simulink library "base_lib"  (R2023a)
settings: Solver=VariableStepAuto  StartTime=0.0  StopTime=10.0  RelTol=1e-3
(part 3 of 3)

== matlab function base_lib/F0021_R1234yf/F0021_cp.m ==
function cp = F0021_cp(T,rho)
%R1234yf_cp
%    CP = R1234yf_cp(T,RHO)

%    This function was generated by the Symbolic Math Toolbox version 9.3.
%    16-Oct-2023 15:47:52

t2 = rho.^2;
t3 = rho.^3;
t5 = rho.^5;
t7 = rho.^7;
t8 = 1.0./T;
t11 = rho./4.17e+3;
t16 = rho.*7.769784172661871e-3;
t24 = rho.*4.892086330935252e-4;
t29 = rho.*2.800959232613909e-3;
t31 = rho.*6.407673860911271e-4;
t32 = rho.*5.059952038369305e-4;
t4 = t2.^2;
t6 = t2.^3;
t9 = t8.^2;
t10 = t8.^3;
t12 = t8.*7.18e+2;
t13 = t8.*8.77e+2;
t14 = t8.*1.755e+3;
t15 = t8.*4.465e+3;
t17 = -t11;
t22 = t8.*5.8856e+4;
t30 = t8.*3.6785e+2;
t33 = t8.*7.94556e+4;
t34 = t2./1.73889e+7;
t39 = t8.*1.044694e+3;
t40 = t11-4.1e+1./2.5e+1;
t48 = t8.*6.54773e+2;
t49 = t8.*1.699467e+3;
t50 = t11-9.1e+1./1.0e+2;
t51 = t11-8.9e+1./1.25e+2;
t52 = t11-3.59e+2./5.0e+2;
t67 = t11-6.77e+2./1.0e+3;
t68 = t16-5.3136e+1;
t77 = t24-1.45248;
t86 = t29-8.38624;
t91 = t31-2.43152;
t99 = t32-1.42847;
t122 = t3.*t8.*9.319180196722149e-10;
t18 = -t12;
t19 = -t13;
t20 = -t14;
t21 = -t15;
t23 = exp(t17);
t41 = -t34;
t42 = t30.^(3.0./2.0);
t43 = t30.^(2.0./5.0);
t44 = t30.^(5.0./2.0);
t45 = t30.^(7.0./2.0);
t46 = t30.^(7.0./5.0);
t53 = t30-6.0./5.0;
t54 = t30.^(1.0./2.0e+1);
t55 = t40.^2;
t56 = t30.^(8.0./2.5e+1);
t58 = t30.^(1.9e+1./2.5e+1);
t60 = t30.^(3.6e+1./2.5e+1);
t61 = t30.^(1.9e+1./5.0e+1);
t62 = t30.^(4.4e+1./2.5e+1);
t64 = t30.^(6.1e+1./2.5e+1);
t65 = t30.^(4.7e+1./5.0e+1);
t66 = t22-2.048e+2;
t69 = t30-3.2e+1./2.5e+1;
t70 = t30-2.3e+1./5.0e+1;
t71 = 1.0./t30.^(3.0./1.0e+2);
t72 = t50.^2;
t73 = t51.^2;
t74 = t52.^2;
t76 = t30.^(9.7e+1./1.0e+2);
t78 = t30-6.7e+1./1.0e+2;
t79 = t30-1.13e+2./1.0e+2;
t80 = t33-2.592e+2;
t81 = t67.^2;
t84 = t30.^(9.29e+2./1.0e+3);
t96 = t39-3.2092;
t102 = t48-8.188e-1;
t105 = t49-3.0954;
t25 = exp(t18);
t26 = exp(t19);
t27 = exp(t20);
t28 = exp(t21);
t47 = exp(t41);
t57 = t54.^21;
t59 = t56.^4;
t63 = t58.^3;
t75 = t53.^2;
t82 = t69.^2;
t83 = t70.^2;
t87 = t78.^2;
t88 = t79.^2;
t89 = t55.*(8.1e+1./5.0);
t94 = t73.*(5.1e+1./5.0e+1);
t98 = t74.*(1.46e+2./2.5e+1);
t100 = t72.*(1.67e+2./1.25e+2);
t106 = t81.*(2.11e+2./2.0e+2);
t114 = t56.*1.546958;
t118 = t84.*2.355237;
t119 = rho.*t65.*2.315508393285372e-4;
t129 = t2.*t61.*3.033007263254145e-8;
t132 = rho.*t23.*t76.*3.263914628297362e-4;
t135 = t2.*t23.*t76.*3.913566700596357e-8;
t35 = t25-1.0;
t36 = t26-1.0;
t37 = t27-1.0;
t38 = t28-1.0;
t85 = t75.*1.08e+2;
t92 = -t89;
t93 = t82.*8.0e+1;
t97 = -t94;
t101 = -t98;
t103 = -t100;
t104 = t83.*(8.9e+1./1.0e+2);
t108 = t88.*(7.1e+1./5.0e+1);
t109 = -t106;
t111 = t87.*(2.31e+2./1.0e+2);
t120 = -t118;
t121 = -t119;
t130 = t47.*t63.*1.210006;
t133 = rho.*t47.*t64.*3.342232613908873e-4;
t136 = t2.*t47.*t63.*1.391699302428561e-7;
t137 = -t135;
t138 = t2.*t47.*t62.*1.06569432224005e-7;
t140 = t3.*t47.*t64.*1.922049476337705e-11;
t141 = t4.*t47.*t62.*4.085726420264459e-15;
t142 = t6.*t23.*t57.*3.588938332192827e-23;
t144 = t7.*t23.*t57.*1.229509534838242e-27;
t90 = -t85;
t95 = -t93;
t107 = -t104;
t110 = -t108;
t112 = -t111;
t131 = -t130;
t134 = -t133;
t139 = -t138;
t143 = -t142;
t113 = t90+t92;
t116 = t95+t101;
t123 = t97+t110;
t125 = t103+t112;
t126 = t107+t109;
t115 = exp(t113);
t117 = exp(t116);
t124 = exp(t123);
t127 = exp(t125);
t128 = exp(t126);
t145 = t2.*t8.*t117.*7.283294189396684e-5;
t147 = rho.*t45.*t115.*1.644384172661871e-7;
t148 = t46.*t124.*1.389966;
t149 = t10.*t127.*2.377824987227386e+7;
t151 = t2.*t45.*t128.*3.407663509480186e-8;
t153 = t3.*t8.*t86.*t117.*5.821977769301905e-9;
t154 = t2.*t45.*t68.*t115.*1.971683660266032e-11;
t156 = rho.*t46.*t77.*t124.*3.333251798561151e-4;
t158 = rho.*t10.*t91.*t127.*5.702218194789895e+3;
t159 = t3.*t45.*t99.*t128.*2.723951646267135e-12;
t146 = -t145;
t150 = -t149;
t152 = -t151;
t155 = -t154;
t157 = -t156;
t160 = t114+t120+t121+t122+t129+t131+t132+t134+t136+t137+t139+t140+t141+t143+t144+t146+t147+t148+t150+t152+t153+t155+t157+t158+t159;
et1 = 1.0./t35.^2.*exp(t8.*-1.436e+3).*2.876052391546904e+1+1.0./t36.^2.*exp(t8.*-1.754e+3).*8.736380352244283+1.0./t37.^2.*exp(t8.*-3.51e+3).*1.696916093943165e+2+1.0./t38.^2.*exp(t8.*-8.93e+3).*2.990869359808914e+2+rho.*t71.^56.*8.072375558752998e-5;
et2 = rho.*1.0./t30.^1.071.*(-3.72539753676259e-5)-(t25.*2.876052391546904e+1)./t35-(t26.*8.736380352244283)./t36-(t27.*1.696916093943165e+2)./t37-(t28.*2.990869359808914e+2)./t38;
et3 = t3.*t71.^54.*5.712042455816759e-13-t2.*1.0./t30.^(5.3e+1./5.0e+1).*1.565883373876438e-9+3.653734124219459e-5./t9+rho.*t30.^(7.0./2.5e+1).*t47.*8.468300984172661e-4;
et4 = rho.*1.0./t54.^12.*t124.*(-1.866621007194245e-4)+t7.*t23.*1.0./t54.^19.*6.454925057900768e-29+t2.*t30.^(1.1e+1./2.5e+1).*t47.*1.408065768852544e-7;
et5 = t3.*t47.*t71.^8.*1.139466607056987e-11+t2.*t23.*1.0./t30.^(1.03e+2./1.0e+2).*1.13884790987354e-9+rho.*t8.*t127.*2.528445291510791e-1;
et6 = rho.*t10.*t127.*(-2.634424805992931e+4)+rho.*t46.*t124.*9.466435107913669e-4-t3.*t8.*t117.*9.315164430883049e-7;
et7 = t2.*t42.*t115.*(-1.725223202732778e-10)+t2.*t45.*t115.*4.258836706174629e-9+t3.*t42.*t128.*2.383457690483743e-11-t3.*t45.*t128.*4.8486339303555e-12;
et8 = t3.*t66.*t117.*(-3.165408600952511e-11)-rho.*t9.*t105.*t127.*9.300886004822446e+1+rho.*t43.*t96.*t124.*9.333105035971223e-4+t2.*t44.*t80.*t115.*1.380178562186222e-10;
et9 = t3.*t44.*t102.*t128.*(-1.906766152386994e-11)+rho.*t10.*t105.^2.*t127.*5.702218194789895e+3-rho.*t46.*t96.^2.*t124.*3.333251798561151e-4;
et10 = t3.*t8.*t66.^2.*t117.*5.821977769301905e-9-t2.*t45.*t80.^2.*t115.*1.971683660266032e-11+t3.*t45.*t102.^2.*t128.*2.723951646267135e-12;
et11 = t65.*9.65567e-1+t137+t144-rho.*t61.*2.529528057553957e-4-t2.*t8.*1.165829442609941e-5-t23.*t76.*1.3610524;
et12 = t47.*t64.*1.393711-t45.*t115.*6.857082e-4+t86.*t153+t91.*t158+t99.*t159+rho.*t23.*t76.*6.527829256594724e-4+rho.*t47.*t62.*8.887890647482015e-4;
et13 = rho.*t47.*t63.*(-1.741015827338129e-3)+rho.*t8.*t117.*6.074267353956834e-1-rho.*t10.*t127.*1.52363270164786e+4+rho.*t46.*t124.*6.799833669064748e-4;
et14 = rho.*t45.*t128.*2.841991366906475e-4+t5.*t23.*t57.*8.979523707146454e-19-t6.*t23.*t57.*7.177876664385654e-23;
et15 = t3.*t47.*t62.*(-1.192623542075196e-10)-t2.*t47.*t64.*4.007473158164116e-7+t3.*t47.*t63.*6.674816798218516e-11+t5.*t47.*t62.*1.95958101691341e-18;
et16 = t4.*t47.*t64.*9.218462716247988e-15-t3.*t8.*t117.*6.800070034544626e-8+t2.*t45.*t115.*6.388255059261943e-10;
et17 = t3.*t45.*t128.*(-5.747537973623655e-12)-t10.*t91.*t127.*4.755649974454772e+7+t46.*t77.*t124.*2.779932+rho.*t45.*t68.*t115.*3.288768345323741e-7;
et18 = t2.*t8.*t86.*t117.*(-1.456658837879337e-4)-t2.*t45.*t99.*t128.*6.815327018960372e-8-rho.*t46.*t77.^2.*t124.*3.333251798561151e-4-t2.*t45.*t68.^2.*t115.*1.971683660266032e-11;
et19 = t3.*2.533418566459739e-12-t47.*t59.*2.75881368-t2.*t117.*1.979963079895795e-7-t9.*t127.*1.93923473200548e+5;
et20 = t43.*t124.*1.9459524+t66.*t145+t80.*t154+t96.*t156+t102.*t151+t105.*t149-rho.*t71.^2.*2.176577889688249e-4+t2.*1.0./t30.^(3.1e+1./5.0e+1).*1.152542760036575e-8+1.0./t30.^(1.7e+1./2.5e+1).*4.9502656e-1;
et21 = 1.0./t30.^(7.1e+1./1.0e+3).*(-2.188015173)+rho.*t23.*t71.*3.165997189448441e-4-rho.*t47.*t60.*8.155047577937649e-4+rho.*t44.*t115.*5.755344604316547e-7;
et22 = t6.*t23.*t54.*(-3.768385248802469e-23)+t7.*t23.*t54.*1.290985011580154e-27-t2.*t23.*t71.*3.796159699578467e-8;
et23 = t2.*t47.*t58.*(-1.875622007142488e-7)+t2.*t47.*t59.*3.173074409537118e-7+t4.*t47.*t58.*7.190878499665448e-15+t3.*t47.*t60.*4.689800722264001e-11;
et24 = t2.*t44.*t128.*(-1.192682228318065e-7)+t3.*t86.*t117.*1.582704300476255e-11-t46.*t96.*t124.*1.389966+rho.*t9.*t91.*t127.*4.650443002411223e+1;
et25 = rho.*t45.*t80.*t115.*(-1.644384172661871e-7)-rho.*t43.*t77.*t124.*4.666552517985612e-4-t2.*t44.*t68.*t115.*6.900892810931111e-11+t3.*t44.*t99.*t128.*9.533830761934972e-12;
et26 = rho.*t10.*t91.*t105.*t127.*(-5.702218194789895e+3)-t3.*t8.*t66.*t86.*t117.*5.821977769301905e-9-t3.*t45.*t99.*t102.*t128.*2.723951646267135e-12;
cp = t9.*(et1+et2+et3+et4+et5+et6+et7+et8+et9+et10).*1.12506132549482e+6+((t11.*t160-rho.*t8.*(et19+et20+et21+et22+et23+et24+et25+et26).*8.821342925659472e-2+1.0).^2.*8.314472)./((rho.*t160)./2.085e+3-(t2.*(et11+et12+et13+et14+et15+et16+et17+et18))./1.73889e+7+1.0);
end

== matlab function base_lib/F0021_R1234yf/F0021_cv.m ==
function cv = F0021_cv(T,rho)
%R1234yf_cv
%    CV = R1234yf_cv(T,RHO)

%    This function was generated by the Symbolic Math Toolbox version 9.3.
%    16-Oct-2023 15:47:50

t2 = rho.^2;
t3 = rho.^3;
t4 = 1.0./T;
t7 = rho./4.17e+3;
t5 = t4.^2;
t6 = t4.^3;
t8 = t4.*7.18e+2;
t9 = t4.*8.77e+2;
t10 = t4.*1.755e+3;
t11 = t4.*4.465e+3;
t12 = -t7;
t17 = t4.*5.8856e+4;
t23 = t4.*3.6785e+2;
t24 = t4.*7.94556e+4;
t25 = t2./1.73889e+7;
t30 = t4.*1.044694e+3;
t31 = t7-4.1e+1./2.5e+1;
t38 = t4.*6.54773e+2;
t39 = t4.*1.699467e+3;
t40 = t7-9.1e+1./1.0e+2;
t41 = t7-8.9e+1./1.25e+2;
t42 = t7-3.59e+2./5.0e+2;
t46 = t7-6.77e+2./1.0e+3;
t13 = -t8;
t14 = -t9;
t15 = -t10;
t16 = -t11;
t18 = exp(t12);
t32 = -t25;
t33 = t23.^(3.0./2.0);
t34 = t23.^(5.0./2.0);
t35 = t23.^(7.0./2.0);
t36 = t23.^(7.0./5.0);
t43 = t23-6.0./5.0;
t44 = t31.^2;
t45 = t17-2.048e+2;
t47 = t23-3.2e+1./2.5e+1;
t48 = t23-2.3e+1./5.0e+1;
t49 = t40.^2;
t50 = t41.^2;
t51 = t42.^2;
t53 = t23-6.7e+1./1.0e+2;
t54 = t23-1.13e+2./1.0e+2;
t55 = t24-2.592e+2;
t56 = t46.^2;
t68 = t30-3.2092;
t73 = t38-8.188e-1;
t76 = t39-3.0954;
t19 = exp(t13);
t20 = exp(t14);
t21 = exp(t15);
t22 = exp(t16);
t37 = exp(t32);
t52 = t43.^2;
t57 = t47.^2;
t58 = t48.^2;
t60 = t53.^2;
t61 = t54.^2;
t62 = t44.*(8.1e+1./5.0);
t66 = t50.*(5.1e+1./5.0e+1);
t70 = t51.*(1.46e+2./2.5e+1);
t71 = t49.*(1.67e+2./1.25e+2);
t77 = t56.*(2.11e+2./2.0e+2);
t26 = t19-1.0;
t27 = t20-1.0;
t28 = t21-1.0;
t29 = t22-1.0;
t59 = t52.*1.08e+2;
t64 = -t62;
t65 = t57.*8.0e+1;
t69 = -t66;
t72 = -t70;
t74 = -t71;
t75 = t58.*(8.9e+1./1.0e+2);
t79 = t61.*(7.1e+1./5.0e+1);
t80 = -t77;
t82 = t60.*(2.31e+2./1.0e+2);
t63 = -t59;
t67 = -t65;
t78 = -t75;
t81 = -t79;
t83 = -t82;
t84 = t63+t64;
t86 = t67+t72;
t88 = t69+t81;
t90 = t74+t83;
t91 = t78+t80;
t85 = exp(t84);
t87 = exp(t86);
t89 = exp(t88);
t92 = exp(t90);
t93 = exp(t91);
et1 = 1.0./t26.^2.*exp(t4.*-1.436e+3).*2.876052391546904e+1+1.0./t27.^2.*exp(t4.*-1.754e+3).*8.736380352244283+1.0./t28.^2.*exp(t4.*-3.51e+3).*1.696916093943165e+2+1.0./t29.^2.*exp(t4.*-8.93e+3).*2.990869359808914e+2+rho.*1.0./t23.^(4.2e+1./2.5e+1).*8.072375558752998e-5;
et2 = rho.*1.0./t23.^1.071.*(-3.72539753676259e-5)-(t19.*2.876052391546904e+1)./t26-(t20.*8.736380352244283)./t27-(t21.*1.696916093943165e+2)./t28-(t22.*2.990869359808914e+2)./t29;
et3 = t2.*1.0./t23.^(5.3e+1./5.0e+1).*(-1.565883373876438e-9)+t3.*1.0./t23.^(8.1e+1./5.0e+1).*5.712042455816759e-13+3.653734124219459e-5./t5+rho.*t23.^(7.0./2.5e+1).*t37.*8.468300984172661e-4;
et4 = rho.*1.0./t23.^(3.0./5.0).*t89.*(-1.866621007194245e-4)+t3.*1.0./t23.^(6.0./2.5e+1).*t37.*1.139466607056987e-11+t2.*t23.^(1.1e+1./2.5e+1).*t37.*1.408065768852544e-7;
et5 = t2.*t18.*1.0./t23.^(1.03e+2./1.0e+2).*1.13884790987354e-9+rho.^7.*t18.*1.0./t23.^(1.9e+1./2.0e+1).*6.454925057900768e-29+rho.*t4.*t92.*2.528445291510791e-1;
et6 = rho.*t6.*t92.*(-2.634424805992931e+4)+rho.*t36.*t89.*9.466435107913669e-4-t3.*t4.*t87.*9.315164430883049e-7;
et7 = t2.*t33.*t85.*(-1.725223202732778e-10)+t2.*t35.*t85.*4.258836706174629e-9+t3.*t33.*t93.*2.383457690483743e-11-t3.*t35.*t93.*4.8486339303555e-12;
et8 = t3.*t45.*t87.*(-3.165408600952511e-11)-rho.*t5.*t76.*t92.*9.300886004822446e+1+t2.*t34.*t55.*t85.*1.380178562186222e-10-t3.*t34.*t73.*t93.*1.906766152386994e-11;
et9 = rho.*t6.*t76.^2.*t92.*5.702218194789895e+3+rho.*t23.^(2.0./5.0).*t68.*t89.*9.333105035971223e-4-rho.*t36.*t68.^2.*t89.*3.333251798561151e-4;
et10 = t3.*t4.*t45.^2.*t87.*5.821977769301905e-9-t2.*t35.*t55.^2.*t85.*1.971683660266032e-11+t3.*t35.*t73.^2.*t93.*2.723951646267135e-12;
cv = t5.*(et1+et2+et3+et4+et5+et6+et7+et8+et9+et10).*1.12506132549482e+6;
end

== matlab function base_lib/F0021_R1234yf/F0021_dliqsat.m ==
function dliq = F0021_dliqsat(T)
% correlation from Martin (1959)


% critical Temp & density
Tc   =     367.85; % [K]
rhoc =     4170.0; % [mol/m3]

T = min(T, Tc);
T = max(T, 0);

% coefficients
x = [   1.768478200876913;
        0.905584244505430;
       -0.353914488877852;
        0.447866446078125 ];

% saturated liquid dfensity
Tr   = T ./ Tc;
A    = [ (1-Tr).^(1/3), (1-Tr).^(2/3), (1-Tr), (1-Tr).^(4/3) ];
dliq = rhoc .* ( 1 + A * x );


end

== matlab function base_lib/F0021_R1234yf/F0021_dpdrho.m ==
function dp_drho = R1234yf_dpdrho(T,rho)
%R1234yf_dpdrho
%    DP_DRHO = R1234yf_dpdrho(T,RHO)

%    This function was generated by the Symbolic Math Toolbox version 9.3.
%    27-Oct-2023 18:05:02

t2 = rho.^2;
t3 = rho.^3;
t5 = rho.^5;
t7 = rho.^7;
t8 = 1.0./T;
t10 = rho./4.17e+3;
t11 = rho.*7.769784172661871e-3;
t14 = rho.*4.892086330935252e-4;
t15 = rho.*2.800959232613909e-3;
t17 = rho.*6.407673860911271e-4;
t18 = rho.*5.059952038369305e-4;
t4 = t2.^2;
t6 = t2.^3;
t9 = t8.^3;
t12 = -t10;
t16 = t8.*3.6785e+2;
t19 = t2./1.73889e+7;
t20 = t10-4.1e+1./2.5e+1;
t25 = t10-9.1e+1./1.0e+2;
t26 = t10-8.9e+1./1.25e+2;
t27 = t10-3.59e+2./5.0e+2;
t36 = t10-6.77e+2./1.0e+3;
t37 = t11-5.3136e+1;
t45 = t14-1.45248;
t52 = t15-8.38624;
t57 = t17-2.43152;
t64 = t18-1.42847;
t13 = exp(t12);
t21 = -t19;
t22 = t16.^(7.0./2.0);
t23 = t16.^(7.0./5.0);
t28 = t16-6.0./5.0;
t29 = t20.^2;
t30 = t16.^(2.1e+1./2.0e+1);
t31 = t16.^(1.9e+1./5.0e+1);
t32 = t16.^(4.4e+1./2.5e+1);
t34 = t16.^(6.1e+1./2.5e+1);
t35 = t16.^(4.7e+1./5.0e+1);
t38 = t16-3.2e+1./2.5e+1;
t39 = t16-2.3e+1./5.0e+1;
t40 = t25.^2;
t41 = t26.^2;
t42 = t27.^2;
t44 = t16.^(9.7e+1./1.0e+2);
t46 = t16-6.7e+1./1.0e+2;
t47 = t16-1.13e+2./1.0e+2;
t48 = t36.^2;
t24 = exp(t21);
t33 = t31.^6;
t43 = t28.^2;
t49 = t38.^2;
t50 = t39.^2;
t53 = t46.^2;
t54 = t47.^2;
t55 = t29.*(8.1e+1./5.0);
t60 = t41.*(5.1e+1./5.0e+1);
t63 = t42.*(1.46e+2./2.5e+1);
t65 = t40.*(1.67e+2./1.25e+2);
t69 = t48.*(2.11e+2./2.0e+2);
t86 = t2.*t13.*t44.*3.913566700596357e-8;
t88 = t7.*t13.*t30.*1.229509534838242e-27;
t51 = t43.*1.08e+2;
t58 = -t55;
t59 = t49.*8.0e+1;
t62 = -t60;
t66 = -t63;
t67 = -t65;
t68 = t50.*(8.9e+1./1.0e+2);
t71 = t54.*(7.1e+1./5.0e+1);
t72 = -t69;
t74 = t53.*(2.31e+2./1.0e+2);
t87 = -t86;
t56 = -t51;
t61 = -t59;
t70 = -t68;
t73 = -t71;
t75 = -t74;
t76 = t56+t58;
t78 = t61+t66;
t80 = t62+t73;
t82 = t67+t75;
t83 = t70+t72;
t77 = exp(t76);
t79 = exp(t78);
t81 = exp(t80);
t84 = exp(t82);
t85 = exp(t83);
et1 = t87+t88-rho.*t35.*2.315508393285372e-4+t3.*t8.*9.319180196722149e-10+t2.*t31.*3.033007263254145e-8-t24.*t33.*1.210006;
et2 = t9.*t84.*(-2.377824987227386e+7)+t23.*t81.*1.389966+t16.^(8.0./2.5e+1).*1.546958-t16.^(9.29e+2./1.0e+3).*2.355237;
et3 = rho.*t13.*t44.*3.263914628297362e-4-rho.*t24.*t34.*3.342232613908873e-4+rho.*t22.*t77.*1.644384172661871e-7-t6.*t13.*t30.*3.588938332192827e-23;
et4 = t2.*t24.*t32.*(-1.06569432224005e-7)+t2.*t24.*t33.*1.391699302428561e-7+t4.*t24.*t32.*4.085726420264459e-15+t3.*t24.*t34.*1.922049476337705e-11;
et5 = t2.*t8.*t79.*(-7.283294189396684e-5)-t2.*t22.*t85.*3.407663509480186e-8-rho.*t23.*t45.*t81.*3.333251798561151e-4+rho.*t9.*t57.*t84.*5.702218194789895e+3;
et6 = t2.*t22.*t37.*t77.*(-1.971683660266032e-11)+t3.*t8.*t52.*t79.*5.821977769301905e-9+t3.*t22.*t64.*t85.*2.723951646267135e-12;
et7 = t35.*9.65567e-1+t87+t88-rho.*t31.*2.529528057553957e-4-t2.*t8.*1.165829442609941e-5-t13.*t44.*1.3610524;
et8 = t24.*t34.*1.393711-t22.*t77.*6.857082e-4+rho.*t24.*t32.*8.887890647482015e-4+rho.*t13.*t44.*6.527829256594724e-4-rho.*t24.*t33.*1.741015827338129e-3;
et9 = rho.*t8.*t79.*6.074267353956834e-1-rho.*t9.*t84.*1.52363270164786e+4+rho.*t23.*t81.*6.799833669064748e-4+rho.*t22.*t85.*2.841991366906475e-4;
et10 = t5.*t13.*t30.*8.979523707146454e-19-t6.*t13.*t30.*7.177876664385654e-23-t3.*t24.*t32.*1.192623542075196e-10;
et11 = t2.*t24.*t34.*(-4.007473158164116e-7)+t3.*t24.*t33.*6.674816798218516e-11+t5.*t24.*t32.*1.95958101691341e-18+t4.*t24.*t34.*9.218462716247988e-15;
et12 = t3.*t8.*t79.*(-6.800070034544626e-8)+t2.*t22.*t77.*6.388255059261943e-10-t3.*t22.*t85.*5.747537973623655e-12+t23.*t45.*t81.*2.779932;
et13 = t9.*t57.*t84.*(-4.755649974454772e+7)+rho.*t22.*t37.*t77.*3.288768345323741e-7-t2.*t8.*t52.*t79.*1.456658837879337e-4-t2.*t22.*t64.*t85.*6.815327018960372e-8;
et14 = rho.*t23.*t45.^2.*t81.*(-3.333251798561151e-4)+rho.*t9.*t57.^2.*t84.*5.702218194789895e+3-t2.*t22.*t37.^2.*t77.*1.971683660266032e-11;
et15 = t3.*t8.*t52.^2.*t79.*5.821977769301905e-9+t3.*t22.*t64.^2.*t85.*2.723951646267135e-12;
dp_drho = T.*((rho.*(et1+et2+et3+et4+et5+et6))./2.085e+3-(t2.*(et7+et8+et9+et10+et11+et12+et13+et14+et15))./1.73889e+7+1.0).*8.314472;
end

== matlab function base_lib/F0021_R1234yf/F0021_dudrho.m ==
function du_drho = R1234yf_dudrho(T,rho)
%R1234yf_dudrho
%    DU_DRHO = R1234yf_dudrho(T,RHO)

%    This function was generated by the Symbolic Math Toolbox version 9.3.
%    19-Oct-2023 14:13:06

t2 = rho.^2;
t3 = rho.^3;
t4 = 1.0./T;
t7 = rho./4.17e+3;
t12 = rho.*1.863257595362559e-6;
t15 = rho.*1.173162189672722e-7;
t19 = rho.*6.716928615381076e-7;
t20 = rho.*1.53661243666937e-7;
t21 = rho.*1.213417755004629e-7;
t5 = t4.^2;
t6 = t4.^3;
t8 = -t7;
t9 = t4.*5.8856e+4;
t11 = t4.*3.6785e+2;
t13 = t4.*7.94556e+4;
t14 = t2./1.73889e+7;
t16 = t4.*1.044694e+3;
t17 = t7-4.1e+1./2.5e+1;
t27 = t4.*6.54773e+2;
t28 = t4.*1.699467e+3;
t29 = t7-9.1e+1./1.0e+2;
t30 = t7-8.9e+1./1.25e+2;
t31 = t7-3.59e+2./5.0e+2;
t39 = t7-6.77e+2./1.0e+3;
t60 = t12-1.274244604316547e-2;
t68 = t15-3.483165467625899e-4;
t79 = t19-2.011088729016787e-3;
t81 = t20-5.830983213429257e-4;
t82 = t21-3.425587529976019e-4;
t10 = exp(t8);
t18 = -t14;
t22 = t11.^(2.0./5.0);
t23 = t11.^(5.0./2.0);
t24 = t11.^(7.0./2.0);
t25 = t11.^(7.0./5.0);
t32 = t11-6.0./5.0;
t33 = t11.^(1.0./2.0e+1);
t34 = t17.^2;
t35 = t11.^(1.9e+1./2.5e+1);
t36 = t11.^(3.2e+1./2.5e+1);
t37 = t11.^(3.6e+1./2.5e+1);
t38 = t9-2.048e+2;
t40 = t11-3.2e+1./2.5e+1;
t41 = t11-2.3e+1./5.0e+1;
t42 = 1.0./t11.^(3.0./1.0e+2);
t43 = t29.^2;
t44 = t30.^2;
t45 = t31.^2;
t47 = t11-6.7e+1./1.0e+2;
t48 = t11-1.13e+2./1.0e+2;
t49 = t13-2.592e+2;
t50 = t39.^2;
t63 = t16-3.2092;
t69 = t27-8.188e-1;
t72 = t28-3.0954;
t26 = exp(t18);
t46 = t32.^2;
t51 = t40.^2;
t52 = t41.^2;
t54 = t47.^2;
t55 = t48.^2;
t56 = t34.*(8.1e+1./5.0);
t61 = t44.*(5.1e+1./5.0e+1);
t65 = t45.*(1.46e+2./2.5e+1);
t66 = t43.*(1.67e+2./1.25e+2);
t73 = t50.*(2.11e+2./2.0e+2);
t53 = t46.*1.08e+2;
t58 = -t56;
t59 = t51.*8.0e+1;
t64 = -t61;
t67 = -t65;
t70 = -t66;
t71 = t52.*(8.9e+1./1.0e+2);
t75 = t55.*(7.1e+1./5.0e+1);
t76 = -t73;
t78 = t54.*(2.31e+2./1.0e+2);
t57 = -t53;
t62 = -t59;
t74 = -t71;
t77 = -t75;
t80 = -t78;
t83 = t57+t58;
t85 = t62+t67;
t87 = t64+t77;
t89 = t70+t80;
t90 = t74+t76;
t84 = exp(t83);
t86 = exp(t85);
t88 = exp(t87);
t91 = exp(t89);
t92 = exp(t90);
et1 = t3.*1.858131002604336e-12-t26.*t36.*2.023446617579852;
et2 = t2.*t86.*(-1.452200134424495e-7)-t5.*t91.*1.422328005554134e+5;
et3 = t22.*t88.*1.427255066297698-rho.*t42.^2.*1.59640689065627e-4;
et4 = t2.*1.0./t11.^(3.1e+1./5.0e+1).*8.453302832006239e-9+1.0./t11.^(1.7e+1./2.5e+1).*3.630762837322852e-1;
et5 = 1.0./t11.^(7.1e+1./1.0e+3).*(-1.60479554422836)+rho.^7.*t10.*t33.*9.468704878352454e-28;
et6 = t2.^3.*t10.*t33.*(-2.763914953991081e-23)+t2.^2.*t26.*t35.*5.274136083584932e-15;
et7 = rho.*t10.*t42.*2.322094583878085e-4-rho.*t26.*t37.*5.981304050145462e-4;
et8 = rho.*t23.*t84.*4.221246493387974e-7-t2.*t10.*t42.*2.784286071796265e-8;
et9 = t2.*t26.*t35.*(-1.37567137415775e-7)+t2.*t26.*t36.*2.327285357417493e-7;
et10 = t3.*t26.*t37.*3.439725370866163e-11-t2.*t23.*t92.*8.74770499448078e-8;
et11 = t3.*t79.*t86.*4.840667114748315e-8+t6.*t72.*t91.*1.74401118947696e+7;
et12 = t25.*t63.*t88.*(-1.019467904498356)-rho.*t24.*t49.*t84.*1.206070426682278e-7;
et13 = rho.*t5.*t81.*t91.*1.422328005554134e+5-rho.*t22.*t68.*t88.*1.427255066297698;
et14 = t2.*t4.*t38.*t86.*5.341918194480503e-5-t2.*t23.*t60.*t84.*2.110623246693987e-7;
et15 = t2.*t24.*t69.*t92.*2.499344284137366e-8+t3.*t23.*t82.*t92.*2.915901664826927e-8;
et16 = rho.*t25.*t63.*t68.*t88.*1.019467904498356-rho.*t6.*t72.*t81.*t91.*1.74401118947696e+7;
et17 = t3.*t4.*t38.*t79.*t86.*(-1.780639398160168e-5)+t2.*t24.*t49.*t60.*t84.*6.030352133411391e-8;
et18 = t3.*t24.*t69.*t82.*t92.*(-8.331147613791219e-9);
du_drho = et1+et2+et3+et4+et5+et6+et7+et8+et9+et10+et11+et12+et13+et14+et15+et16+et17+et18;
end

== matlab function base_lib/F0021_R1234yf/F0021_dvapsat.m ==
function dvap = F0021_dvapsat(T)

% critical Temp & density
Tc   =     367.85; % [K]
% rhoc =     4170.0; % [mol/m3]

T = min(T, Tc);
T = max(T, 0);

% coefficients
x = [ 8.5116; -7.9050; 1.6189; 2.6394; -1.3847 ];

% saturated vapor density
Tr   = T ./ Tc;
th   = 1 ./ (1 - Tr);
A    = [ ones(size(Tr)), log(th).^(-1.5), log(th).^(-2), log(th).^(-3), log(th).^(-4) ];
dvap = exp(A*x);


end

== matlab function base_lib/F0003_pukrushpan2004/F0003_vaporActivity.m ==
function a = F0003_vaporActivity(p, P_sat)
a = p ./ P_sat; % [-] - water vapor activity
end

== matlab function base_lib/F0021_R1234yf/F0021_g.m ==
function g = F0021_g(T,rho)
%R1234yf_g
%    G = R1234yf_g(T,RHO)

%    This function was generated by the Symbolic Math Toolbox version 9.3.
%    16-Oct-2023 15:47:52

t2 = rho.^2;
t3 = rho.^3;
t5 = rho.^7;
t6 = 1.0./T;
t8 = rho./4.17e+3;
t4 = t2.^2;
t7 = t6.^3;
t9 = -t8;
t11 = t6.*3.6785e+2;
t12 = t2./1.73889e+7;
t13 = t8-4.1e+1./2.5e+1;
t18 = t8-9.1e+1./1.0e+2;
t19 = t8-8.9e+1./1.25e+2;
t20 = t8-3.59e+2./5.0e+2;
t30 = t8-6.77e+2./1.0e+3;
t10 = exp(t9);
t14 = -t12;
t15 = t11.^(7.0./2.0);
t16 = t11.^(7.0./5.0);
t21 = t11-6.0./5.0;
t22 = t13.^2;
t23 = t11.^(8.0./2.5e+1);
t24 = t11.^(2.1e+1./2.0e+1);
t25 = t11.^(1.9e+1./5.0e+1);
t26 = t11.^(4.4e+1./2.5e+1);
t28 = t11.^(6.1e+1./2.5e+1);
t29 = t11.^(4.7e+1./5.0e+1);
t31 = t11-3.2e+1./2.5e+1;
t32 = t11-2.3e+1./5.0e+1;
t33 = t18.^2;
t34 = t19.^2;
t35 = t20.^2;
t37 = t11.^(9.7e+1./1.0e+2);
t38 = t11-6.7e+1./1.0e+2;
t39 = t11-1.13e+2./1.0e+2;
t40 = t30.^2;
t43 = t11.^(9.29e+2./1.0e+3);
t17 = exp(t14);
t27 = t25.^6;
t36 = t21.^2;
t41 = t31.^2;
t42 = t32.^2;
t45 = t38.^2;
t46 = t39.^2;
t47 = t22.*(8.1e+1./5.0);
t51 = t34.*(5.1e+1./5.0e+1);
t54 = t35.*(1.46e+2./2.5e+1);
t55 = t33.*(1.67e+2./1.25e+2);
t59 = t40.*(2.11e+2./2.0e+2);
t76 = t2.*t10.*t37.*3.913566700596357e-8;
t77 = t5.*t10.*t24.*1.229509534838242e-27;
t44 = t36.*1.08e+2;
t49 = -t47;
t50 = t41.*8.0e+1;
t53 = -t51;
t56 = -t54;
t57 = -t55;
t58 = t42.*(8.9e+1./1.0e+2);
t61 = t46.*(7.1e+1./5.0e+1);
t62 = -t59;
t64 = t45.*(2.31e+2./1.0e+2);
t48 = -t44;
t52 = -t50;
t60 = -t58;
t63 = -t61;
t65 = -t64;
t66 = t48+t49;
t68 = t52+t56;
t70 = t53+t63;
t72 = t57+t65;
t73 = t60+t62;
t67 = exp(t66);
t69 = exp(t68);
t71 = exp(t70);
t74 = exp(t72);
t75 = exp(t73);
et1 = t23.*1.546958-t43.*2.355237-t76+t77-rho.*t29.*2.315508393285372e-4+t3.*t6.*9.319180196722149e-10;
et2 = t2.*t25.*3.033007263254145e-8-t17.*t27.*1.210006-t7.*t74.*2.377824987227386e+7+t16.*t71.*1.389966;
et3 = t2.^3.*t10.*t24.*(-3.588938332192827e-23)-rho.*t17.*t28.*3.342232613908873e-4+rho.*t10.*t37.*3.263914628297362e-4+rho.*t15.*t67.*1.644384172661871e-7;
et4 = t2.*t17.*t26.*(-1.06569432224005e-7)+t2.*t17.*t27.*1.391699302428561e-7+t4.*t17.*t26.*4.085726420264459e-15+t3.*t17.*t28.*1.922049476337705e-11;
et5 = t2.*t6.*t69.*(-7.283294189396684e-5)-t2.*t15.*t75.*3.407663509480186e-8-rho.*t16.*t71.*(rho.*4.892086330935252e-4-1.45248).*3.333251798561151e-4;
et6 = rho.*t7.*t74.*(rho.*6.407673860911271e-4-2.43152).*5.702218194789895e+3-t2.*t15.*t67.*(rho.*7.769784172661871e-3-5.3136e+1).*1.971683660266032e-11;
et7 = t3.*t6.*t69.*(rho.*2.800959232613909e-3-8.38624).*5.821977769301905e-9+t3.*t15.*t75.*(rho.*5.059952038369305e-4-1.42847).*2.723951646267135e-12;
et8 = t6.*2.95847224925e+3+t76-t77+log(-exp(t6.*-7.18e+2)+1.0).*7.549+log(-exp(t6.*-8.77e+2)+1.0).*1.537+log(-exp(t6.*-1.755e+3)+1.0).*7.455+log(-exp(t6.*-4.465e+3)+1.0).*(2.03e+2./1.0e+2)+log(t8)+log(t11).*(6.18e+2./1.25e+2)+rho.*t23.*3.709731414868106e-4;
et9 = rho.*t43.*(-5.64805035971223e-4)+t4.*t6.*5.587038487243495e-14+t3.*t25.*2.424466237613225e-12-t2.*t29.*2.776388960773827e-8+t8.*(et1+et2+et3+et4+et5+et6+et7);
et10 = rho.*t17.*t27.*(-2.901693045563549e-4)-rho.*t7.*t74.*5.702218194789895e+3+rho.*t16.*t71.*3.333251798561151e-4-t3.*t17.*t26.*8.518739586251397e-12;
et11 = t2.*t17.*t28.*(-4.007473158164116e-8)-t3.*t6.*t69.*5.821977769301905e-9+t2.*t15.*t67.*1.971683660266032e-11-t3.*t15.*t75.*2.723951646267135e-12;
et12 = -1.1837928e+1;
g = T.*(et8+et9+et10+et11+et12).*8.314472;
end

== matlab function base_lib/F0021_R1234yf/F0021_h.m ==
function h = F0021_h(T,rho)
%R1234yf_h
%    H = R1234yf_h(T,RHO)

%    This function was generated by the Symbolic Math Toolbox version 9.3.
%    16-Oct-2023 15:47:51

t2 = rho.^2;
t3 = rho.^3;
t5 = rho.^7;
t6 = 1.0./T;
t8 = rho./4.17e+3;
t4 = t2.^2;
t7 = t6.^3;
t9 = t6.*7.18e+2;
t10 = t6.*8.77e+2;
t11 = t6.*1.755e+3;
t12 = t6.*4.465e+3;
t13 = -t8;
t23 = t6.*3.6785e+2;
t24 = t2./1.73889e+7;
t25 = t8-4.1e+1./2.5e+1;
t31 = t8-9.1e+1./1.0e+2;
t32 = t8-8.9e+1./1.25e+2;
t33 = t8-3.59e+2./5.0e+2;
t40 = t8-6.77e+2./1.0e+3;
t14 = -t9;
t15 = -t10;
t16 = -t11;
t17 = -t12;
t18 = exp(t13);
t26 = -t24;
t27 = t23.^(5.0./2.0);
t28 = t23.^(7.0./2.0);
t29 = t23.^(7.0./5.0);
t34 = t23-6.0./5.0;
t35 = t25.^2;
t36 = t23.^(2.1e+1./2.0e+1);
t37 = t23.^(4.4e+1./2.5e+1);
t38 = t23.^(5.7e+1./2.5e+1);
t39 = t23.^(6.1e+1./2.5e+1);
t41 = t23-3.2e+1./2.5e+1;
t42 = t23-2.3e+1./5.0e+1;
t43 = t31.^2;
t44 = t32.^2;
t45 = t33.^2;
t47 = t23.^(9.7e+1./1.0e+2);
t48 = t23-6.7e+1./1.0e+2;
t49 = t23-1.13e+2./1.0e+2;
t50 = t40.^2;
t19 = exp(t14);
t20 = exp(t15);
t21 = exp(t16);
t22 = exp(t17);
t30 = exp(t26);
t46 = t34.^2;
t51 = t41.^2;
t52 = t42.^2;
t54 = t48.^2;
t55 = t49.^2;
t56 = t35.*(8.1e+1./5.0);
t60 = t44.*(5.1e+1./5.0e+1);
t63 = t45.*(1.46e+2./2.5e+1);
t64 = t43.*(1.67e+2./1.25e+2);
t68 = t50.*(2.11e+2./2.0e+2);
t53 = t46.*1.08e+2;
t58 = -t56;
t59 = t51.*8.0e+1;
t62 = -t60;
t65 = -t63;
t66 = -t64;
t67 = t52.*(8.9e+1./1.0e+2);
t70 = t55.*(7.1e+1./5.0e+1);
t71 = -t68;
t73 = t54.*(2.31e+2./1.0e+2);
t57 = -t53;
t61 = -t59;
t69 = -t67;
t72 = -t70;
t74 = -t73;
t75 = t57+t58;
t77 = t61+t65;
t79 = t62+t72;
t81 = t66+t74;
t82 = t69+t71;
t76 = exp(t75);
t78 = exp(t77);
t80 = exp(t79);
t83 = exp(t81);
t84 = exp(t82);
et1 = T.*(-1.344026097594128e-2)-t4.*1.518836071019028e-16+(t19.*1.473476145167867e+1)./(t19-1.0)+(t20.*3.66439853201033)./(t20-1.0)+(t21.*3.556755470980019e+1)./(t21-1.0)+(t22.*2.464034253092293e+1)./(t22-1.0)+t3.*t78.*1.582704300476255e-11;
et2 = rho.*1.0./t23.^(1.7e+1./2.5e+1).*(-1.187114052757794e-4)+rho.*1.0./t23.^(7.1e+1./1.0e+3).*5.247038784172661e-4+t2.*1.0./t23.^(3.0./5.0e+1).*2.609805623127397e-8;
et3 = t3.*1.0./t23.^(3.1e+1./5.0e+1).*(-9.212971702930256e-13)+rho.*t6.^2.*t83.*4.650443002411223e+1-rho.*t23.^(2.0./5.0).*t80.*4.666552517985612e-4;
et4 = rho.*t23.^(3.2e+1./2.5e+1).*t30.*6.615860143884892e-4+t5.*t18.*t23.^(1.0./2.0e+1).*1.290985011580154e-27+t3.*t23.^(1.9e+1./2.5e+1).*t30.*1.499298167180246e-11;
et5 = t2.*t23.^(3.6e+1./2.5e+1).*t30.*9.778234505920443e-8-t2.*t18.*1.0./t23.^(3.0./1.0e+2).*3.796159699578467e-8-t2.*t27.*t76.*6.900892810931111e-11;
et6 = t3.*t27.*t84.*9.533830761934972e-12+rho.*t29.*t80.*(t6.*1.044694e+3-3.2092).*3.333251798561151e-4-rho.*t7.*t83.*(t6.*1.699467e+3-3.0954).*5.702218194789895e+3;
et7 = t3.*t6.*t78.*(t6.*5.8856e+4-2.048e+2).*(-5.821977769301905e-9)+t2.*t28.*t76.*(t6.*7.94556e+4-2.592e+2).*1.971683660266032e-11;
et8 = t3.*t28.*t84.*(t6.*6.54773e+2-8.188e-1).*(-2.723951646267135e-12)-8.042605;
et9 = t3.*t6.*9.319180196722149e-10-t30.*t38.*1.210006-t7.*t83.*2.377824987227386e+7+t29.*t80.*1.389966;
et10 = rho.*t23.^(4.7e+1./5.0e+1).*(-2.315508393285372e-4)+t2.*t23.^(1.9e+1./5.0e+1).*3.033007263254145e-8+t23.^(8.0./2.5e+1).*1.546958-t23.^(9.29e+2./1.0e+3).*2.355237;
et11 = t2.^3.*t18.*t36.*(-3.588938332192827e-23)+rho.*t18.*t47.*3.263914628297362e-4-rho.*t30.*t39.*3.342232613908873e-4+rho.*t28.*t76.*1.644384172661871e-7;
et12 = t5.*t18.*t36.*1.229509534838242e-27-t2.*t18.*t47.*3.913566700596357e-8-t2.*t30.*t37.*1.06569432224005e-7+t2.*t30.*t38.*1.391699302428561e-7;
et13 = t4.*t30.*t37.*4.085726420264459e-15+t3.*t30.*t39.*1.922049476337705e-11-t2.*t6.*t78.*7.283294189396684e-5-t2.*t28.*t84.*3.407663509480186e-8;
et14 = rho.*t29.*t80.*(rho.*4.892086330935252e-4-1.45248).*(-3.333251798561151e-4)+rho.*t7.*t83.*(rho.*6.407673860911271e-4-2.43152).*5.702218194789895e+3;
et15 = t2.*t28.*t76.*(rho.*7.769784172661871e-3-5.3136e+1).*(-1.971683660266032e-11)+t3.*t6.*t78.*(rho.*2.800959232613909e-3-8.38624).*5.821977769301905e-9;
et16 = t3.*t28.*t84.*(rho.*5.059952038369305e-4-1.42847).*2.723951646267135e-12;
h = T.*(t6.*(et1+et2+et3+et4+et5+et6+et7+et8).*(-3.6785e+2)+t8.*(et9+et10+et11+et12+et13+et14+et15+et16)+1.0).*8.314472;
end

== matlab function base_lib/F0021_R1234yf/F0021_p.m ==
function p = F0021_p(T,rho)
%R1234yf_p
%    P = R1234yf_p(T,RHO)

%    This function was generated by the Symbolic Math Toolbox version 9.3.
%    16-Oct-2023 15:47:49

t2 = rho.^2;
t3 = rho.^3;
t4 = 1.0./T;
t6 = rho./4.17e+3;
t5 = t4.^3;
t7 = -t6;
t9 = t4.*3.6785e+2;
t10 = t2./1.73889e+7;
t11 = t6-4.1e+1./2.5e+1;
t16 = t6-9.1e+1./1.0e+2;
t17 = t6-8.9e+1./1.25e+2;
t18 = t6-3.59e+2./5.0e+2;
t25 = t6-6.77e+2./1.0e+3;
t8 = exp(t7);
t12 = -t10;
t13 = t9.^(7.0./2.0);
t14 = t9.^(7.0./5.0);
t19 = t9-6.0./5.0;
t20 = t11.^2;
t21 = t9.^(2.1e+1./2.0e+1);
t22 = t9.^(4.4e+1./2.5e+1);
t23 = t9.^(5.7e+1./2.5e+1);
t24 = t9.^(6.1e+1./2.5e+1);
t26 = t9-3.2e+1./2.5e+1;
t27 = t9-2.3e+1./5.0e+1;
t28 = t16.^2;
t29 = t17.^2;
t30 = t18.^2;
t32 = t9.^(9.7e+1./1.0e+2);
t33 = t9-6.7e+1./1.0e+2;
t34 = t9-1.13e+2./1.0e+2;
t35 = t25.^2;
t15 = exp(t12);
t31 = t19.^2;
t36 = t26.^2;
t37 = t27.^2;
t39 = t33.^2;
t40 = t34.^2;
t41 = t20.*(8.1e+1./5.0);
t45 = t29.*(5.1e+1./5.0e+1);
t48 = t30.*(1.46e+2./2.5e+1);
t49 = t28.*(1.67e+2./1.25e+2);
t53 = t35.*(2.11e+2./2.0e+2);
t38 = t31.*1.08e+2;
t43 = -t41;
t44 = t36.*8.0e+1;
t47 = -t45;
t50 = -t48;
t51 = -t49;
t52 = t37.*(8.9e+1./1.0e+2);
t55 = t40.*(7.1e+1./5.0e+1);
t56 = -t53;
t58 = t39.*(2.31e+2./1.0e+2);
t42 = -t38;
t46 = -t44;
t54 = -t52;
t57 = -t55;
t59 = -t58;
t60 = t42+t43;
t62 = t46+t50;
t64 = t47+t57;
t66 = t51+t59;
t67 = t54+t56;
t61 = exp(t60);
t63 = exp(t62);
t65 = exp(t64);
t68 = exp(t66);
t69 = exp(t67);
et1 = t3.*t4.*9.319180196722149e-10-t15.*t23.*1.210006-t5.*t68.*2.377824987227386e+7+t14.*t65.*1.389966;
et2 = rho.*t9.^(4.7e+1./5.0e+1).*(-2.315508393285372e-4)+t2.*t9.^(1.9e+1./5.0e+1).*3.033007263254145e-8+t9.^(8.0./2.5e+1).*1.546958-t9.^(9.29e+2./1.0e+3).*2.355237;
et3 = rho.^7.*t8.*t21.*1.229509534838242e-27-t2.^3.*t8.*t21.*3.588938332192827e-23+t2.^2.*t15.*t22.*4.085726420264459e-15;
et4 = rho.*t15.*t24.*(-3.342232613908873e-4)+rho.*t8.*t32.*3.263914628297362e-4+rho.*t13.*t61.*1.644384172661871e-7-t2.*t15.*t22.*1.06569432224005e-7;
et5 = t2.*t15.*t23.*1.391699302428561e-7-t2.*t8.*t32.*3.913566700596357e-8+t3.*t15.*t24.*1.922049476337705e-11-t2.*t4.*t63.*7.283294189396684e-5;
et6 = t2.*t13.*t69.*(-3.407663509480186e-8)-rho.*t14.*t65.*(rho.*4.892086330935252e-4-1.45248).*3.333251798561151e-4+rho.*t5.*t68.*(rho.*6.407673860911271e-4-2.43152).*5.702218194789895e+3;
et7 = t2.*t13.*t61.*(rho.*7.769784172661871e-3-5.3136e+1).*(-1.971683660266032e-11)+t3.*t4.*t63.*(rho.*2.800959232613909e-3-8.38624).*5.821977769301905e-9;
et8 = t3.*t13.*t69.*(rho.*5.059952038369305e-4-1.42847).*2.723951646267135e-12;
p = T.*rho.*(t6.*(et1+et2+et3+et4+et5+et6+et7+et8)+1.0).*8.314472;
end

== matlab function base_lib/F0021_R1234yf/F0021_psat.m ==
function p_sat = F0021_psat(T)
% Van Laar, J. L Res Tray Chim 39 (1920) 21
% fit to data from 
% Richter, Mclinden, Lemmon Journal of. Chem. E (2011)

% critical Temp & density
Tc   =     367.85; % [K]

T = max(T,0);
T = min(T, Tc);


% R1234yf coefficients
n = [ -4.893666065312787; 
       0.111013414194105; 
       0.000025221844863;
       -0.015565681357114] * 1e3;

% saturation pressure
p_sat = exp( n(1) .* (1./T) + n(2) + n(3) .* T + n(4) .* log(T) ); 
end

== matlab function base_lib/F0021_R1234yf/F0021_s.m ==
function s = F0021_s(T,rho)
%R1234yf_s
%    S = R1234yf_s(T,RHO)

%    This function was generated by the Symbolic Math Toolbox version 9.3.
%    16-Oct-2023 15:47:49

t2 = rho.^2;
t3 = rho.^3;
t5 = rho.^7;
t6 = 1.0./T;
t8 = rho./4.17e+3;
t4 = t2.^2;
t7 = t6.^3;
t9 = t6.*7.18e+2;
t10 = t6.*8.77e+2;
t11 = t6.*1.755e+3;
t12 = t6.*4.465e+3;
t13 = -t8;
t23 = t6.*3.6785e+2;
t24 = t2./1.73889e+7;
t25 = t8-4.1e+1./2.5e+1;
t31 = t8-9.1e+1./1.0e+2;
t32 = t8-8.9e+1./1.25e+2;
t33 = t8-3.59e+2./5.0e+2;
t36 = t8-6.77e+2./1.0e+3;
t14 = -t9;
t15 = -t10;
t16 = -t11;
t17 = -t12;
t18 = exp(t13);
t26 = -t24;
t27 = t23.^(5.0./2.0);
t28 = t23.^(7.0./2.0);
t29 = t23.^(7.0./5.0);
t34 = t23-6.0./5.0;
t35 = t25.^2;
t37 = t23-3.2e+1./2.5e+1;
t38 = t23-2.3e+1./5.0e+1;
t39 = t31.^2;
t40 = t32.^2;
t41 = t33.^2;
t43 = t23-6.7e+1./1.0e+2;
t44 = t23-1.13e+2./1.0e+2;
t45 = t36.^2;
t19 = exp(t14);
t20 = exp(t15);
t21 = exp(t16);
t22 = exp(t17);
t30 = exp(t26);
t42 = t34.^2;
t46 = t37.^2;
t47 = t38.^2;
t49 = t43.^2;
t50 = t44.^2;
t51 = t35.*(8.1e+1./5.0);
t55 = t40.*(5.1e+1./5.0e+1);
t58 = t41.*(1.46e+2./2.5e+1);
t59 = t39.*(1.67e+2./1.25e+2);
t63 = t45.*(2.11e+2./2.0e+2);
t48 = t42.*1.08e+2;
t53 = -t51;
t54 = t46.*8.0e+1;
t57 = -t55;
t60 = -t58;
t61 = -t59;
t62 = t47.*(8.9e+1./1.0e+2);
t65 = t50.*(7.1e+1./5.0e+1);
t66 = -t63;
t68 = t49.*(2.31e+2./1.0e+2);
t52 = -t48;
t56 = -t54;
t64 = -t62;
t67 = -t65;
t69 = -t68;
t70 = t52+t53;
t72 = t56+t60;
t74 = t57+t67;
t76 = t61+t69;
t77 = t64+t66;
t71 = exp(t70);
t73 = exp(t72);
t75 = exp(t74);
t78 = exp(t76);
t79 = exp(t77);
et1 = T.*(-1.344026097594128e-2)-t4.*1.518836071019028e-16+(t19.*1.473476145167867e+1)./(t19-1.0)+(t20.*3.66439853201033)./(t20-1.0)+(t21.*3.556755470980019e+1)./(t21-1.0)+(t22.*2.464034253092293e+1)./(t22-1.0)+t3.*t73.*1.582704300476255e-11;
et2 = rho.*1.0./t23.^(1.7e+1./2.5e+1).*(-1.187114052757794e-4)+rho.*1.0./t23.^(7.1e+1./1.0e+3).*5.247038784172661e-4+t2.*1.0./t23.^(3.0./5.0e+1).*2.609805623127397e-8;
et3 = t3.*1.0./t23.^(3.1e+1./5.0e+1).*(-9.212971702930256e-13)+rho.*t6.^2.*t78.*4.650443002411223e+1-rho.*t23.^(2.0./5.0).*t75.*4.666552517985612e-4;
et4 = rho.*t23.^(3.2e+1./2.5e+1).*t30.*6.615860143884892e-4+t5.*t18.*t23.^(1.0./2.0e+1).*1.290985011580154e-27+t3.*t23.^(1.9e+1./2.5e+1).*t30.*1.499298167180246e-11;
et5 = t2.*t23.^(3.6e+1./2.5e+1).*t30.*9.778234505920443e-8-t2.*t18.*1.0./t23.^(3.0./1.0e+2).*3.796159699578467e-8-t2.*t27.*t71.*6.900892810931111e-11;
et6 = t3.*t27.*t79.*9.533830761934972e-12+rho.*t29.*t75.*(t6.*1.044694e+3-3.2092).*3.333251798561151e-4-rho.*t7.*t78.*(t6.*1.699467e+3-3.0954).*5.702218194789895e+3;
et7 = t3.*t6.*t73.*(t6.*5.8856e+4-2.048e+2).*(-5.821977769301905e-9)+t2.*t28.*t71.*(t6.*7.94556e+4-2.592e+2).*1.971683660266032e-11;
et8 = t3.*t28.*t79.*(t6.*6.54773e+2-8.188e-1).*(-2.723951646267135e-12)-8.042605;
et9 = t6.*(-2.459813467916615e+4)-log(-t19+1.0).*6.2765949128e+1-log(-t20+1.0).*1.2779343464e+1;
et10 = log(-t21+1.0).*(-6.198438876e+1)-log(-t22+1.0).*1.687837816e+1-log(t8).*8.314472-log(t23).*4.1106749568e+1;
et11 = t4.*t6.*(-4.64532750651084e-13)-t6.*(et1+et2+et3+et4+et5+et6+et7+et8).*3.0584785252e+3;
et12 = rho.*t23.^(8.0./2.5e+1).*(-3.084445797644125e-3)+rho.*t23.^(9.29e+2./1.0e+3).*4.696055657041726e-3;
et13 = t3.*t23.^(1.9e+1./5.0e+1).*(-2.015815664758051e-11)+t2.*t23.^(4.7e+1./5.0e+1).*2.308420827546308e-7;
et14 = rho.*t23.^(5.7e+1./2.5e+1).*t30.*2.412604557993285e-3+t5.*t18.*t23.^(2.1e+1./2.0e+1).*1.022272260114558e-26;
et15 = t3.*t23.^(4.4e+1./2.5e+1).*t30.*7.082882176517883e-11+t2.*t23.^(6.1e+1./2.5e+1).*t30.*3.332002336430711e-7;
et16 = t2.*t18.*t23.^(9.7e+1./1.0e+2).*(-3.25392407522408e-7)+rho.*t7.*t78.*4.741093351847113e+4;
et17 = rho.*t29.*t75.*(-2.771422874808633e-3)+t3.*t6.*t73.*4.840667114748315e-8;
et18 = t2.*t28.*t71.*(-1.639350858613943e-10)+t3.*t28.*t79.*2.2648219692242e-11;
et19 = 1.06740592894016e+2;
s = et9+et10+et11+et12+et13+et14+et15+et16+et17+et18+et19;
end

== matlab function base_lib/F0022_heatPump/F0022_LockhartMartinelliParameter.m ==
function X_tt = F0022_LockhartMartinelliParameter(x, rho_g, rho_f, mu_g, mu_f)

% Lockhart-Martinelly Parameter (nuclear-power.com)
X_tt = ((1-x)./x).^0.9 .* (rho_g ./ rho_f).^0.5 .* (mu_f ./ mu_g ).^0.1;


end

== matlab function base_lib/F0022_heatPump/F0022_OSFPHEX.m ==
function h = F0022_OSFPHEX(G, x, rho_f, rho_g, cp_f, cp_g, mu_f, mu_g, k_f, k_g, sigma, par)

% parameters
D_h = par.D_h;

% output size
h = zeros(size(x));

% Bond number
g   = 9.81;
B_d = g .* (rho_f - rho_g) .* D_h.^2 ./ sigma;

% liquid & gas Prandtl number
Pr_f = cp_f .* mu_f ./ k_f;
Pr_g = cp_g .* mu_g ./ k_g;

% minimum mass flux
G = max(G, 1);

% refrigerant side heat transfer coefficient
G_eq  = G .* ( (1-x) + (rho_f./rho_g).^0.5 .* x );
Re_f  = G    .* D_h ./ mu_f;
Re_g  = G    .* D_h ./ mu_g;
Re_eq = G_eq .* D_h ./ mu_f;
Nu    = 3.918 .* Re_eq.^0.505 .* Re_f.^(-0.1354) .* B_d.^0.213 .* Pr_f.^(1/3);
h_tp     = Nu .* k_f ./ D_h;

% single phase correlation
h_f = 0.494 .* G .* cp_f .* Re_f.^(-0.426) .* Pr_f.^(-2/3);
h_g = 0.494 .* G .* cp_g .* Re_g.^(-0.426) .* Pr_g.^(-2/3);

% smooth transition to subcooled liquid & superheated vapor
y = (x-0.1) / 0.1;
y = tanh(y*5)/2 + 1/2;
z =  (x-0.90) / 0.1;
z = tanh(z*5)/2 + 1/2;

h = h_tp .* y .* (1-z) + h_f .* (1-y) + h_g .* z;

% output
% h       = h_tp;
% h(x==0) = h_f(x==0);
% h(x==1) = h_g(x==1);



end

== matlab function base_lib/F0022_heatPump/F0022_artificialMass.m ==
function m = F0022_artificialMass(p, par)

% parameters
B       = par.BV .* par.V;
rho_ref = par.rho_ref;
V       = par.V;

% artificial mass
m = V .* rho_ref .* (p./B + 1);


end

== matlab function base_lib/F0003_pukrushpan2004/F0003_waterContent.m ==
function lambda = F0003_waterContent(a)
lambda = zeros(length(a),1);
lambda( a <= 1) = 0.043 + 17.81.*a - 39.85.*a.^2 + 36.*a.^3;
lambda( a > 1)  = 14 + 1.4*(a-1);
end

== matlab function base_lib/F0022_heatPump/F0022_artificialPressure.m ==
function p = F0022_artificialPressure(m, par)

% parameters
V = par.V;
B = par.BV .* par.V;
rho_ref = par.rho_ref;


% artificial pressure
p = B .* (m./(V .* rho_ref) - 1); 

end

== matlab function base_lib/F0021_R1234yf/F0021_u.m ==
function u = F0021_u(T,rho)
%R1234yf_u
%    U = R1234yf_u(T,RHO)

%    This function was generated by the Symbolic Math Toolbox version 9.3.
%    16-Oct-2023 15:47:50

t2 = rho.^2;
t3 = rho.^3;
t4 = 1.0./T;
t5 = rho./4.17e+3;
t6 = t4.*7.18e+2;
t7 = t4.*8.77e+2;
t8 = t4.*1.755e+3;
t9 = t4.*4.465e+3;
t10 = -t5;
t20 = t4.*3.6785e+2;
t21 = t2./1.73889e+7;
t22 = t5-4.1e+1./2.5e+1;
t27 = t5-9.1e+1./1.0e+2;
t28 = t5-8.9e+1./1.25e+2;
t29 = t5-3.59e+2./5.0e+2;
t32 = t5-6.77e+2./1.0e+3;
t11 = -t6;
t12 = -t7;
t13 = -t8;
t14 = -t9;
t15 = exp(t10);
t23 = -t21;
t24 = t20.^(5.0./2.0);
t25 = t20.^(7.0./2.0);
t30 = t20-6.0./5.0;
t31 = t22.^2;
t33 = t20-3.2e+1./2.5e+1;
t34 = t20-2.3e+1./5.0e+1;
t35 = t27.^2;
t36 = t28.^2;
t37 = t29.^2;
t39 = t20-6.7e+1./1.0e+2;
t40 = t20-1.13e+2./1.0e+2;
t41 = t32.^2;
t16 = exp(t11);
t17 = exp(t12);
t18 = exp(t13);
t19 = exp(t14);
t26 = exp(t23);
t38 = t30.^2;
t42 = t33.^2;
t43 = t34.^2;
t45 = t39.^2;
t46 = t40.^2;
t47 = t31.*(8.1e+1./5.0);
t51 = t36.*(5.1e+1./5.0e+1);
t54 = t37.*(1.46e+2./2.5e+1);
t55 = t35.*(1.67e+2./1.25e+2);
t59 = t41.*(2.11e+2./2.0e+2);
t44 = t38.*1.08e+2;
t49 = -t47;
t50 = t42.*8.0e+1;
t53 = -t51;
t56 = -t54;
t57 = -t55;
t58 = t43.*(8.9e+1./1.0e+2);
t61 = t46.*(7.1e+1./5.0e+1);
t62 = -t59;
t64 = t45.*(2.31e+2./1.0e+2);
t48 = -t44;
t52 = -t50;
t60 = -t58;
t63 = -t61;
t65 = -t64;
t66 = t48+t49;
t68 = t52+t56;
t70 = t53+t63;
t72 = t57+t65;
t73 = t60+t62;
t67 = exp(t66);
t69 = exp(t68);
t71 = exp(t70);
t74 = exp(t72);
t75 = exp(t73);
et1 = T.*4.1106749568e+1-(t16.*4.5065951473904e+4)./(t16-1.0)-(t17.*1.1207484217928e+4)./(t17-1.0)-(t18.*1.087826022738e+5)./(t18-1.0);
et2 = (t19.*(-7.53619584844e+4))./(t19-1.0)-t3.*t69.*4.840667114748315e-8;
et3 = rho.*1.0./t20.^(1.7e+1./2.5e+1).*3.630762837322852e-1-rho.*1.0./t20.^(7.1e+1./1.0e+3).*1.60479554422836;
et4 = t2.*1.0./t20.^(3.0./5.0e+1).*(-7.982034453281349e-5)+t3.*1.0./t20.^(3.1e+1./5.0e+1).*2.817767610668746e-9;
et5 = t2.^2.*4.64532750651084e-13-rho.*t4.^2.*t74.*1.422328005554134e+5;
et6 = rho.*t20.^(2.0./5.0).*t71.*1.427255066297698-rho.*t20.^(3.2e+1./2.5e+1).*t26.*2.023446617579852;
et7 = t3.*t20.^(1.9e+1./2.5e+1).*t26.*(-4.585571247192502e-8)-t2.*t20.^(3.6e+1./2.5e+1).*t26.*2.990652025072731e-4;
et8 = t2.*t15.*1.0./t20.^(3.0./1.0e+2).*1.161047291939042e-4-rho.^7.*t15.*t20.^(1.0./2.0e+1).*3.948449934272973e-24;
et9 = t2.*t24.*t67.*2.110623246693987e-7-t3.*t24.*t75.*2.915901664826927e-8;
et10 = rho.*t20.^(7.0./5.0).*t71.*(t4.*1.044694e+3-3.2092).*(-1.019467904498356);
et11 = rho.*t4.^3.*t74.*(t4.*1.699467e+3-3.0954).*1.74401118947696e+7;
et12 = t3.*t4.*t69.*(t4.*5.8856e+4-2.048e+2).*1.780639398160168e-5-t2.*t25.*t67.*(t4.*7.94556e+4-2.592e+2).*6.030352133411391e-8;
et13 = t3.*t25.*t75.*(t4.*6.54773e+2-8.188e-1).*8.331147613791219e-9+2.459813467916615e+4;
u = et1+et2+et3+et4+et5+et6+et7+et8+et9+et10+et11+et12+et13;
end

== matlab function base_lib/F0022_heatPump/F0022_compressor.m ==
function [m_dot, P_cmp, h_2]  = F0022_compressor(p_1, rho_1, h_1, p_2, N, k, par)
% model from Li 2013

% parameters
V_disp = par.V_disp; 
N_ref  = par.N_ref / 60;
M      = par.M;

% M = 0.1140415928; % [kg/mol]  compressor displacement
% V_disp = 0.00017; % [m3]   compressor displacement
% N_ref = 2000 / 60; % [rps]  reference speed

% suction properties
p_s   = p_1;
rho_s = rho_1;
h_s   = h_1;

% discharge properties
p_d = p_2;

% compressor parameters
b1    = 0.799;
b2    = -0.036;
a1    = 1.140;
a2    = 0.295;
a3    = 447.050;
Wloss = 350.000;
d1    = 1.223;
d2    = -0.206;
d3    = -0.017;
e1    = 0.507;
e2    = 0.606;
e3    = -0.113;

% reference volumetric efficieny
nv_ref = b1 + b2 .* (  (p_d./p_s ).^(1./k) );

% reference volume flow
dV_ref = nv_ref .* N_ref .* V_disp;

% reference compressor power
P_ref = p_s .* dV_ref .* a1 .* ( (p_d./p_s).^(a2 + (k-1)./k) + a3./p_d ) + Wloss; 

% volumetric efficiency ratio
nv = d1 + d2 .* (N./N_ref) + d3 .* (N./N_ref).^2;

% isentropic efficiency ratio
ni = e1 + e2 .* (N./N_ref) + e3 .* (N./N_ref).^2; 

% Compressor suction volume flow
dV_suc = dV_ref .* (N./N_ref) .* nv;
m_dot  = dV_suc  .* rho_s .* M;

% Compressor power
P_cmp = P_ref .* dV_suc ./ dV_ref .* ni;

% discharge enthalpy
h_d = M.* P_cmp ./ (m_dot + 1e-5) + h_s;
h_2 = h_d;

end

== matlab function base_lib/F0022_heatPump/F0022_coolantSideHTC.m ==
function h = F0022_coolantSideHTC(G, par)
% parameters
mu = par.mu_clt;
k  = par.k_clt;
cp = par.cp_clt;

G = max(1,G);

% hydraulic diameter
D_h = par.D_h;

% Reynolds number
Re = G .* D_h ./ mu;

% Prandtl number
Pr = cp .* mu ./ k;

% HTC
h = 0.494 .* G .* cp .* Re.^(-0.426) .* Pr.^(-2/3);

end

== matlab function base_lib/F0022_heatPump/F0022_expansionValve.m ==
function dp = F0022_expansionValve(W, p_us, T_us, rho_us, T_sat, alpha, par)

% parameters
M  = par.M;
Tc = par.Tc;
D  = par.D;

% constants
R = 8.314472;

% exv geometry
A = alpha .* D.^2 .* pi / 4;

% degree of subcooling
T_sub = max(T_sat - T_us, 0);

% flow coefficient
a  = [ 0.7568; -1.7428; 1.0530; 2.2342; 2.9406;  -8.4168 ];
AA = [ones(size(p_us)), alpha, alpha.^2, alpha .* T_sub/Tc, T_sub/Tc,  (T_sub/Tc).^2 ];
C  = AA * a;

% pressure drop
dp =  1./rho_us .*  (W ./ (C.*A)).^2;


% pressure drop
% dp = p_us - p_ds;

% flow
% W = C.*A .* sqrt( rho_us .* max(dp,0) );

end

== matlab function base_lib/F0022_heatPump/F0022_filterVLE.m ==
function B = F0022_filterVLE(B, B_liq, B_vap, x)

% assign saturated property
B( x > 0 & x < 1) = x .* B_vap + (1-x) .* B_liq;


end

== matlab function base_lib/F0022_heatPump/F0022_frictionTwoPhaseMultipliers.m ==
function [Phi_Ltt, Phi_Gtt] = F0022_frictionTwoPhaseMultipliers(X_tt, Re)


% Liquid
Phi_Ltt = 1 + C./X_tt + 1./X_tt.^2;

% Gas
Phi_Gtt = 1 + C.*X_tt + X_tt.^2;



end

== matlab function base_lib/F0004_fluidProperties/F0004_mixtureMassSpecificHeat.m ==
function [cp, cv] = F0004_mixtureMassSpecificHeat(p, par)
% total pressure
p_tot = sum(p);

% mass specific heat capacity
cp_r  = par.cp_r;
cp_v  = par.cp_H2O;
cp_N2 = par.cp_N2;
R_r    = par.R_r;
R_H2O  = par.R_H2O;
R_N2   = par.R_N2;

% partial pressures
p_r  = p(1);
p_v  = p(2);
p_N2 = p(3);

% mole fractions
x_r   = p_r  ./ p_tot;
x_v   = p_v  ./ p_tot;
x_N2  = p_N2 ./ p_tot;

% average mass
M_avg = sum([x_r, x_v, x_N2] .* [par.M_r, par.M_H2O, par.M_N2]);

% mole fraction to mass fraction
w_r   = x_r  .* par.M_r   ./ M_avg;
w_v   = x_v  .* par.M_H2O ./ M_avg;
w_N2  = x_N2 .* par.M_N2  ./ M_avg;

% mixture gas constant
Rm = w_r.*R_r + w_v.*R_H2O + w_N2 .* R_N2;

% ideal mixture heat capacity
cp = w_r.*cp_r + w_v.*cp_v + w_N2 .* cp_N2;
cv = cp - Rm;

end

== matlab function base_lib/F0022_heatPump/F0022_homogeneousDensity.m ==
function rho_H = F0022_homogeneousDensity(x, rho_f, rho_g)

% thermopedia.com /cn/content/37/
rho_h = rho_f .* rho_g ./ ( x.* rho_f + (1-x) .* rho_g );

end

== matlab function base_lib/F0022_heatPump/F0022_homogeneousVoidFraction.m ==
function e = F0022_homogeneousVoidFraction(x, rho_liq, rho_vap)

% from Engineering Data Book II, Wolverine Tube Inc.

e = 1 ./ ( 1 + (1-x)./x .* rho_vap ./ rho_liq );


end
